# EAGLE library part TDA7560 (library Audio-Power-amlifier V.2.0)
The TDA7560 is a breakthrough BCD (Bipolar / CMOS / DMOS) technology class AB Audio Power Amplifier in Flexiwatt 25 package designed for high power car radio. The fully complementary P-Channel/N-Channel output structure allows a rail to rail output voltage swing which, combined with high output current and minimised saturation losses sets new power references in the car-radio field, with unparalleled distortion performances.
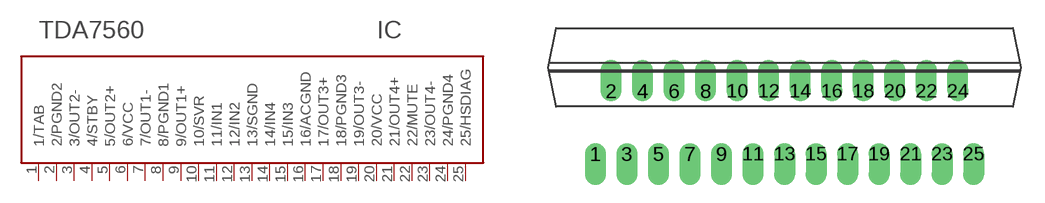
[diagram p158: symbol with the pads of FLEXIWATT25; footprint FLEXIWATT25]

Designator prefix IC

## TDA7560  [FLEXIWATT25]
1  1/TAB
2  2/PGND2  pwr
3  3/OUT2-  out
4  4/STBY  in
5  5/OUT2+  out
6  6/VCC  pwr
7  7/OUT1-  out
8  8/PGND1  pwr
9  9/OUT1+  out
10  10/SVR
11  11/IN1  in
12  12/IN2  in
13  13/SGND  pwr
14  14/IN4  in
15  15/IN3  in
16  16/ACGND  pwr
17  17/OUT3+  out
18  18/PGND3  pwr
19  19/OUT3-  out
20  20/VCC  pwr
21  21/OUT4+  out
22  22/MUTE  in
23  23/OUT4-  out
24  24/PGND4  pwr
25  25/HSDIAG  in

## Footprint FLEXIWATT25 (pad centres in mm)
Flexiwatt25 (vertical)
drill 0.813 offset: 1 -12,0; 2 -11,4; 3 -10,0; 4 -9,4; 5 -8,0; 6 -7,4; 7 -6,0; 8 -5,4; 9 -4,0; 10 -3,4; 11 -2,0; 12 -1,4; 13 0,0; 14 1,4; 15 2,0; 16 3,4; 17 4,0; 18 5,4; 19 6,0; 20 7,4; 21 8,0; 22 9,4; 23 10,0; 24 11,4; 25 12,0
